(* Logix 5000 AddOnInstructionDefinition export SPEL_XYLimSet; software revision 30.01 *)

ADD_ON_INSTRUCTION SPEL_ExecCmd   (* revision 1.2 *)
// Executes a command in the robot controller.  Normally this is called by higher level AOIs.
VAR_INPUT
   Start : BOOL; {required}
   MaxTime : DINT := 3000; {required}
END_VAR
VAR_OUTPUT
   InCycle : BOOL; {access Read Only, visible}
   Done : BOOL; {access Read Only, visible}
   Error : BOOL; {access Read Only, visible}
END_VAR
VAR_IN_OUT
   ExtInputs : AB:ETHERNET_MODULE_INT_128Bytes:I:0; {required}
        .DATA[0].0   // ExtCmdGet
        .DATA[0].1   // ExtRespSet
        .DATA[0].2   // ExtCmdResult
        .DATA[0].3   // ExtError
   ExtOutputs : AB:ETHERNET_MODULE_INT_128Bytes:O:0; {required}
        .DATA[0].0   // ExtCmdSet
        .DATA[0].1   // ExtRespGet
        .DATA[0].2   // ExtCmdReset
END_VAR
VAR_INPUT
   Cmd : INT; {required}
   CmdParam1 : INT; {required}
   CmdParam2 : INT; {required}
   CmdParam3 : INT; {required}
   CmdParam4 : INT; {required}
   CmdParam5 : INT; {required}
   CmdParam6 : INT; {required}
   CmdParam7 : INT; {required}
END_VAR
VAR_OUTPUT
   CmdEcho : INT; {access Read Only, visible}
   Resp1 : INT; {access Read Only, visible}
   Resp2 : INT; {access Read Only, visible}
   Resp3 : INT; {access Read Only, visible}
   Resp4 : INT; {access Read Only, visible}
   Resp5 : INT; {access Read Only, visible}
   Resp6 : INT; {access Read Only, visible}
   Resp7 : INT; {access Read Only, visible}
   ErrCode1 : INT; {access Read Only, visible}
   ErrCode2 : INT; {access Read Only, visible}
END_VAR
VAR
   ExtReset : BOOL; {access None}
   ExtError : BOOL; {access None}
   ExtCmdSet : BOOL; {access None}   // Cmd Ready
   ExtCmdGet : BOOL; {access None}   // Cmd Received
   CmdXferDone : BOOL; {access None}
   ExtRespSet : BOOL; {access None}   // Resp Ready
   RespXferDone : BOOL; {access None}
   ExtCmdResult : BOOL; {access None}   // Normal or Error?
   TmrCmdDataRdy : TIMER := (PRE := 5); {access None}
   OneShotDoneOff : BOOL; {access None}
   OneShotStart : BOOL; {access None}
   StartInit : BOOL; {access None}
   OneShotStartError : BOOL; {access None}
   TmrCycle : TIMER := (PRE := 5000); {access None}
   OneshotTmrPreset : BOOL; {access None}
   TmrCmdSet : TIMER := (PRE := 20); {access None}
   OnShotCmdDataXfer : BOOL; {access None}
   OneShotRespDataXfer : BOOL; {access None}
   OneShotDataRdy : BOOL; {access None}
   OtherCmdInCycle : BOOL; {access None}
   s : BOOL; {access None}
   OneShotUnsetCmdIncycle : BOOL; {access None}
   OneShotSetCmdIncycle : BOOL; {access None}
   OneShotSetOtherCmdInCycleError : BOOL; {access None}
   OneShotSetBit : BOOL; {access None}
   MaxTimeError : BOOL; {access None}
END_VAR

ROUTINE Logic   (* ladder *)
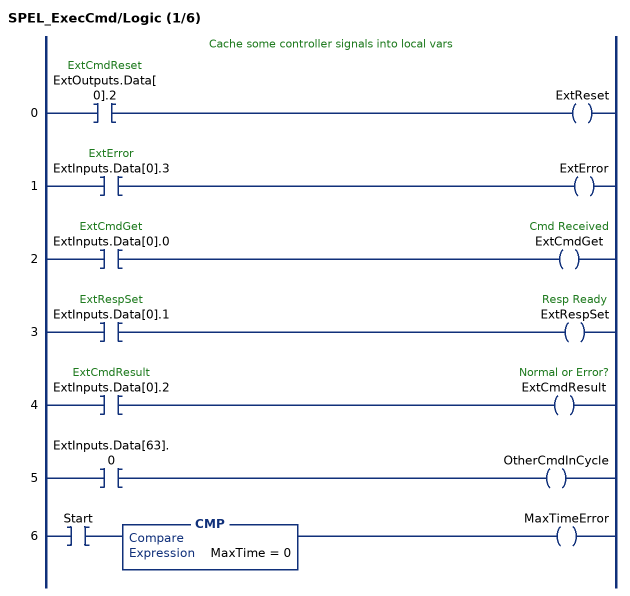
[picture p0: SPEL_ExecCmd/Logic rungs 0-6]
   // Cache some controller signals into local vars
   0: XIC(ExtOutputs.Data[0].2)OTE(ExtReset);
   1: XIC(ExtInputs.Data[0].3)OTE(ExtError);
   2: XIC(ExtInputs.Data[0].0)OTE(ExtCmdGet);
   3: XIC(ExtInputs.Data[0].1)OTE(ExtRespSet);
   4: XIC(ExtInputs.Data[0].2)OTE(ExtCmdResult);
   5: XIC(ExtInputs.Data[63].0)OTE(OtherCmdInCycle);
   6: XIC(Start)CMP(MaxTime = 0)OTE(MaxTimeError);
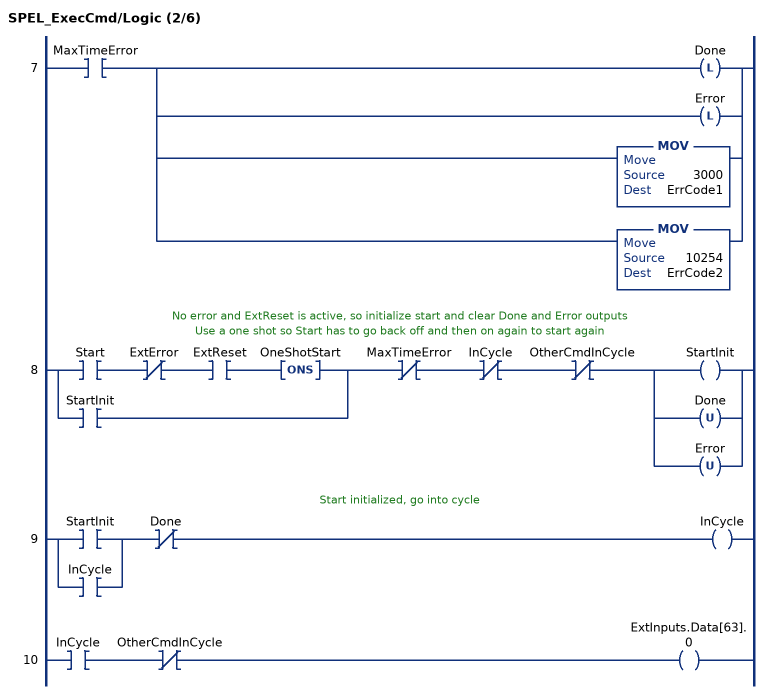
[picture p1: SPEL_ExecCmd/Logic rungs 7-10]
   7: XIC(MaxTimeError)[OTL(Done) ,OTL(Error) ,MOV(3000,ErrCode1) ,MOV(10254,ErrCode2) ];
   // No error and ExtReset is active, so initialize start and clear Done and Error outputs
   // Use a one shot so Start has to go back off and then on again to start again
   8: [XIC(Start) XIO(ExtError) XIC(ExtReset) ONS(OneShotStart) ,XIC(StartInit) ]XIO(MaxTimeError)XIO(InCycle)XIO(OtherCmdInCycle)[OTE(StartInit) ,OTU(Done) ,OTU(Error) ];
   // Start initialized, go into cycle
   9: [XIC(StartInit) ,XIC(InCycle) ]XIO(Done)OTE(InCycle);
   10: XIC(InCycle)XIO(OtherCmdInCycle)OTE(ExtInputs.Data[63].0);
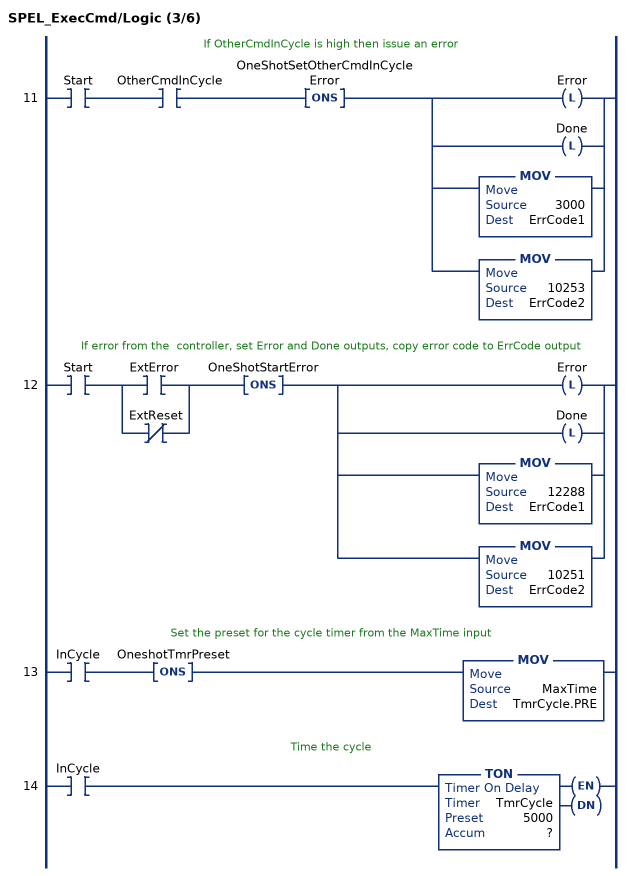
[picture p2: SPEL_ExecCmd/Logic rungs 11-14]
   // If OtherCmdInCycle is high then issue an error
   11: XIC(Start)XIC(OtherCmdInCycle)ONS(OneShotSetOtherCmdInCycleError)[OTL(Error) ,OTL(Done) ,MOV(3000,ErrCode1) ,MOV(10253,ErrCode2) ];
   // If error from the  controller, set Error and Done outputs, copy error code to ErrCode output
   12: XIC(Start)[XIC(ExtError) ,XIO(ExtReset) ]ONS(OneShotStartError)[OTL(Error) ,OTL(Done) ,MOV(12288,ErrCode1) ,MOV(10251,ErrCode2) ];
   // Set the preset for the cycle timer from the MaxTime input
   13: XIC(InCycle)ONS(OneshotTmrPreset)MOV(MaxTime,TmrCycle.PRE);
   // Time the cycle
   14: XIC(InCycle)TON(TmrCycle,?,?);
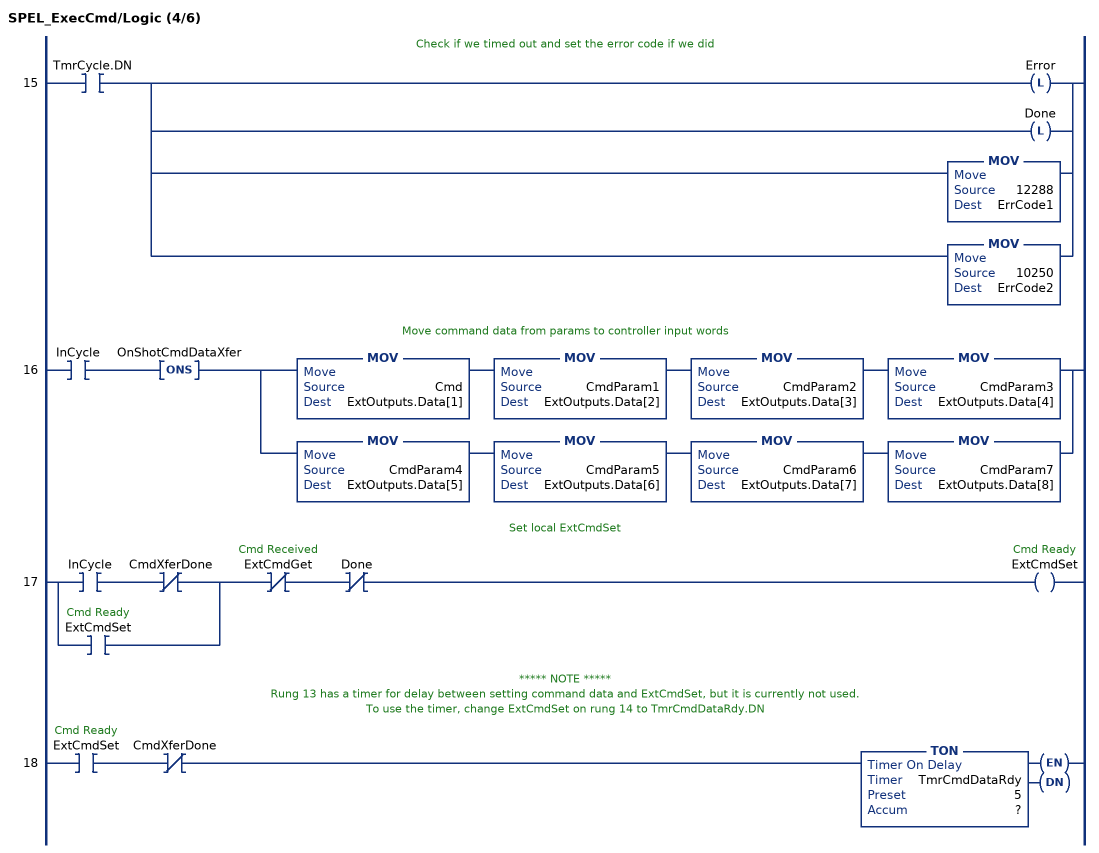
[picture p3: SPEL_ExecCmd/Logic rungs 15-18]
   // Check if we timed out and set the error code if we did
   15: XIC(TmrCycle.DN)[OTL(Error) ,OTL(Done) ,MOV(12288,ErrCode1) ,MOV(10250,ErrCode2) ];
   // Move command data from params to controller input words
   16: XIC(InCycle)ONS(OnShotCmdDataXfer)[MOV(Cmd,ExtOutputs.Data[1]) MOV(CmdParam1,ExtOutputs.Data[2]) MOV(CmdParam2,ExtOutputs.Data[3]) MOV(CmdParam3,ExtOutputs.Data[4]) ,MOV(CmdParam4,ExtOutputs.Data[5]) MOV(CmdParam5,ExtOutputs.Data[6]) MOV(CmdParam6,ExtOutputs.Data[7]) MOV(CmdParam7,ExtOutputs.Data[8]) ];
   // Set local ExtCmdSet
   17: [XIC(InCycle) XIO(CmdXferDone) ,XIC(ExtCmdSet) ]XIO(ExtCmdGet)XIO(Done)OTE(ExtCmdSet);
   // ***** NOTE *****
   // Rung 13 has a timer for delay between setting command data and ExtCmdSet, but it is currently not used.
   // To use the timer, change ExtCmdSet on rung 14 to TmrCmdDataRdy.DN
   18: XIC(ExtCmdSet)XIO(CmdXferDone)TON(TmrCmdDataRdy,?,?);
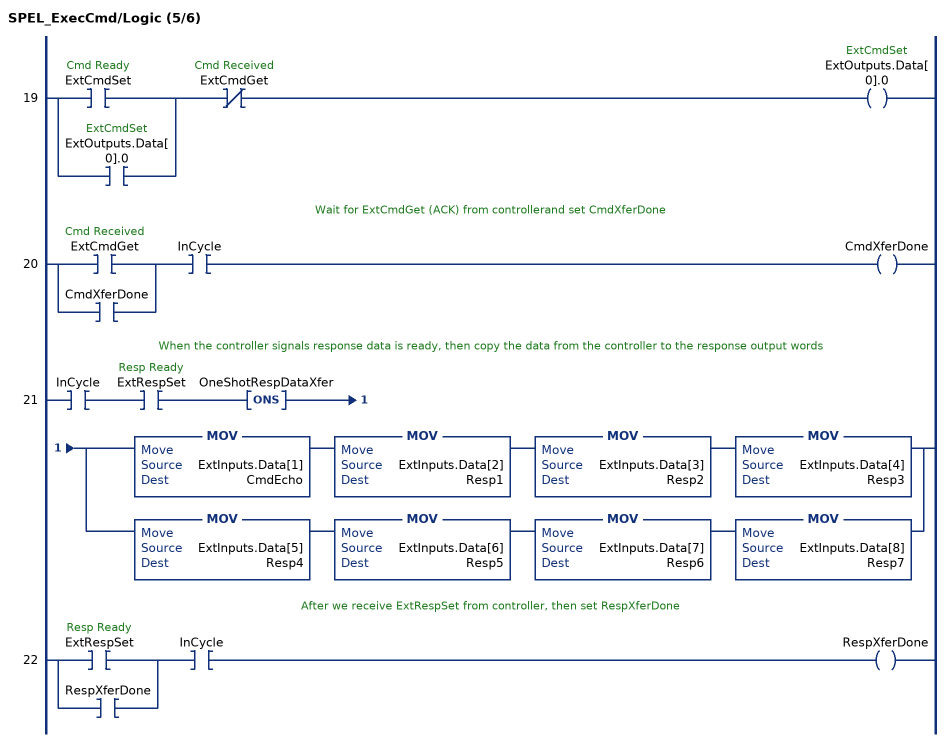
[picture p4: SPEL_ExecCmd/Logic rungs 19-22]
   19: [XIC(ExtCmdSet) ,XIC(ExtOutputs.Data[0].0) ]XIO(ExtCmdGet)OTE(ExtOutputs.Data[0].0);
   // Wait for ExtCmdGet (ACK) from controllerand set CmdXferDone
   20: [XIC(ExtCmdGet) ,XIC(CmdXferDone) ]XIC(InCycle)OTE(CmdXferDone);
   // When the controller signals response data is ready, then copy the data from the controller to the response output words
   21: XIC(InCycle)XIC(ExtRespSet)ONS(OneShotRespDataXfer)[MOV(ExtInputs.Data[1],CmdEcho) MOV(ExtInputs.Data[2],Resp1) MOV(ExtInputs.Data[3],Resp2) MOV(ExtInputs.Data[4],Resp3) ,MOV(ExtInputs.Data[5],Resp4) MOV(ExtInputs.Data[6],Resp5) MOV(ExtInputs.Data[7],Resp6) MOV(ExtInputs.Data[8],Resp7) ];
   // After we receive ExtRespSet from controller, then set RespXferDone
   22: [XIC(ExtRespSet) ,XIC(RespXferDone) ]XIC(InCycle)OTE(RespXferDone);
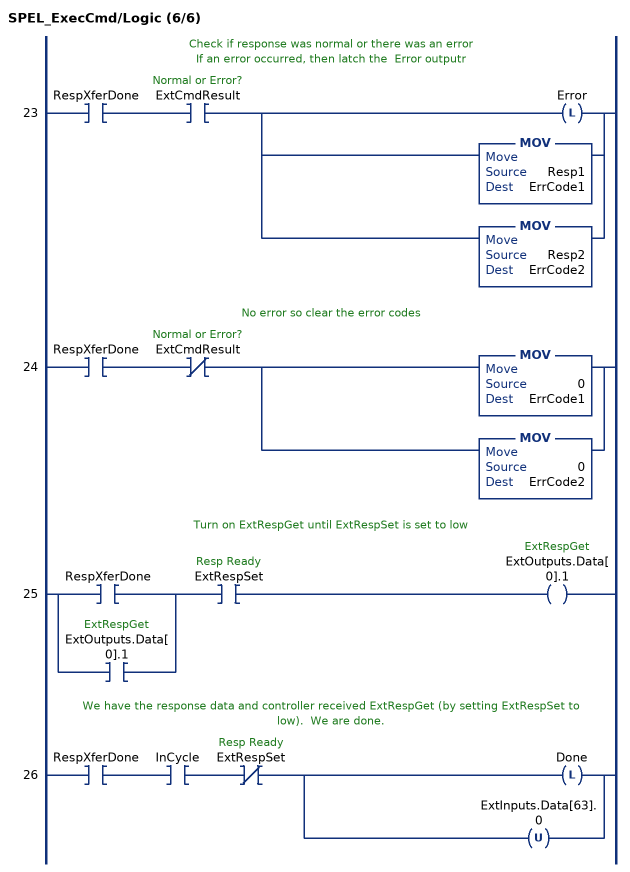
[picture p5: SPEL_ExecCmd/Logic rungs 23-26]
   // Check if response was normal or there was an error
   // If an error occurred, then latch the  Error outputr
   23: XIC(RespXferDone)XIC(ExtCmdResult)[OTL(Error) ,MOV(Resp1,ErrCode1) ,MOV(Resp2,ErrCode2) ];
   // No error so clear the error codes
   24: XIC(RespXferDone)XIO(ExtCmdResult)[MOV(0,ErrCode1) ,MOV(0,ErrCode2) ];
   // Turn on ExtRespGet until ExtRespSet is set to low
   25: [XIC(RespXferDone) ,XIC(ExtOutputs.Data[0].1) ]XIC(ExtRespSet)OTE(ExtOutputs.Data[0].1);
   // We have the response data and controller received ExtRespGet (by setting ExtRespSet to low).  We are done.
   26: XIC(RespXferDone)XIC(InCycle)XIO(ExtRespSet)[OTL(Done) ,OTU(ExtInputs.Data[63].0) ];
END_ROUTINE
END_ADD_ON_INSTRUCTION

ADD_ON_INSTRUCTION SPEL_XYLimSet   (* revision 1.2, vendor SEIKO EPSON CORP. *)
// Sets the allowable motion area by specifying the
// lower and upper limit positions.
VAR_OUTPUT
   InCycle : BOOL; {access Read Only, visible}
   Done : BOOL; {access Read Only, visible}
   Error : BOOL; {access Read Only, visible}
END_VAR
VAR_INPUT
   Start : BOOL; {required}
   XLower : REAL; {access Read Only, required}
   XUpper : REAL; {access Read Only, required}
   YLower : REAL; {access Read Only, required}
   YUpper : REAL; {access Read Only, required}
   ZLower : REAL; {access Read Only, required}
   ZUpper : REAL; {access Read Only, required}
END_VAR
VAR_IN_OUT
   ExtInputs : AB:ETHERNET_MODULE_INT_128Bytes:I:0; {required}
   ExtOutputs : AB:ETHERNET_MODULE_INT_128Bytes:O:0; {required}
END_VAR
VAR_OUTPUT
   ErrCode1 : INT; {access Read Only, visible}
   ErrCode2 : INT; {access Read Only, visible}
END_VAR
VAR
   ExecXYLimSetZ : SPEL_ExecCmd := (MaxTime := 3000); {access None}
   ExecXYLimSetY : SPEL_ExecCmd := (MaxTime := 3000); {access None}
   ExecXYLimSetX : SPEL_ExecCmd := (MaxTime := 3000); {access None}
   upperLimit_INTS : INT[2]; {access None}
   StartInit : BOOL[32]; {access None}
   OneShotStart : BOOL[32]; {access None}
   lowerLimit_INTS : INT[2]; {access None}
   Lowerx1000 : DINT; {access None}
   Upperx1000 : DINT; {access None}
   ExecTimeout : DINT; {access None}
END_VAR

ROUTINE Logic   (* ladder *)
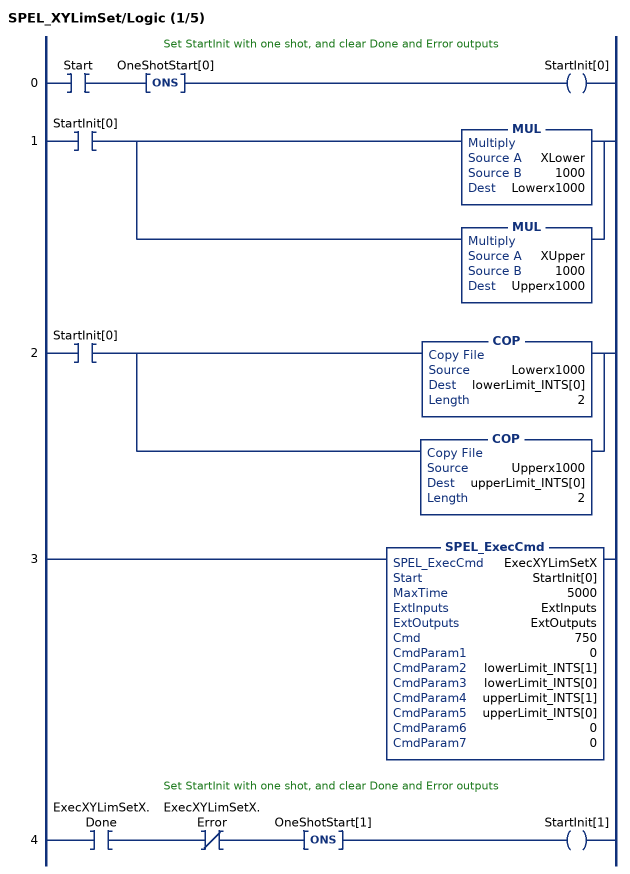
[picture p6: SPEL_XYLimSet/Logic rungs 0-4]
   // Set StartInit with one shot, and clear Done and Error outputs
   0: XIC(Start)ONS(OneShotStart[0])OTE(StartInit[0]);
   1: XIC(StartInit[0])[MUL(XLower,1000,Lowerx1000) ,MUL(XUpper,1000,Upperx1000) ];
   2: XIC(StartInit[0])[COP(Lowerx1000,lowerLimit_INTS[0],2) ,COP(Upperx1000,upperLimit_INTS[0],2) ];
   3: SPEL_ExecCmd(ExecXYLimSetX,StartInit[0],5000,ExtInputs,ExtOutputs,750,0,lowerLimit_INTS[1],lowerLimit_INTS[0],upperLimit_INTS[1],upperLimit_INTS[0],0,0);
   // Set StartInit with one shot, and clear Done and Error outputs
   4: XIC(ExecXYLimSetX.Done)XIO(ExecXYLimSetX.Error)ONS(OneShotStart[1])OTE(StartInit[1]);
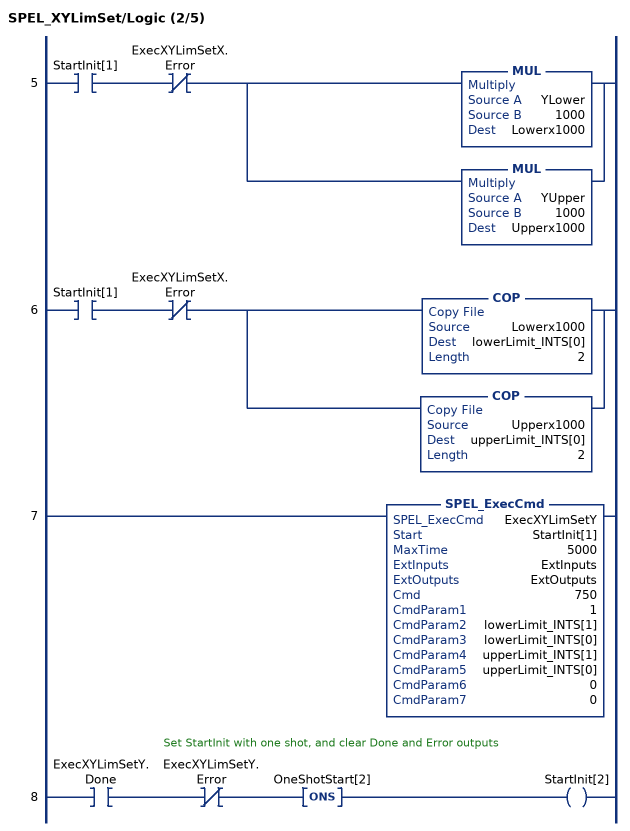
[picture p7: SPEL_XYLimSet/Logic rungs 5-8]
   5: XIC(StartInit[1])XIO(ExecXYLimSetX.Error)[MUL(YLower,1000,Lowerx1000) ,MUL(YUpper,1000,Upperx1000) ];
   6: XIC(StartInit[1])XIO(ExecXYLimSetX.Error)[COP(Lowerx1000,lowerLimit_INTS[0],2) ,COP(Upperx1000,upperLimit_INTS[0],2) ];
   7: SPEL_ExecCmd(ExecXYLimSetY,StartInit[1],5000,ExtInputs,ExtOutputs,750,1,lowerLimit_INTS[1],lowerLimit_INTS[0],upperLimit_INTS[1],upperLimit_INTS[0],0,0);
   // Set StartInit with one shot, and clear Done and Error outputs
   8: XIC(ExecXYLimSetY.Done)XIO(ExecXYLimSetY.Error)ONS(OneShotStart[2])OTE(StartInit[2]);
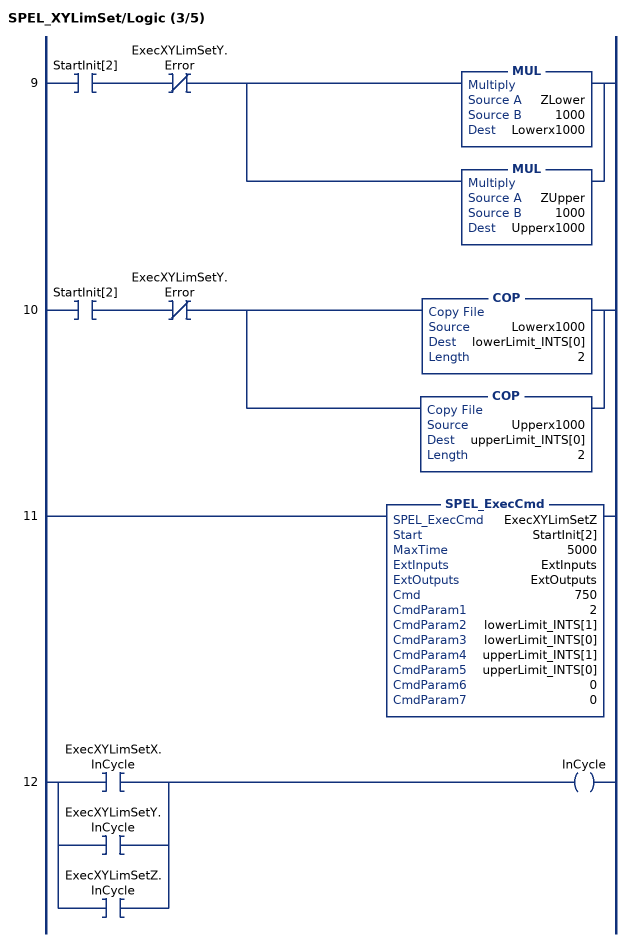
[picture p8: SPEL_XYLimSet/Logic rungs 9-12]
   9: XIC(StartInit[2])XIO(ExecXYLimSetY.Error)[MUL(ZLower,1000,Lowerx1000) ,MUL(ZUpper,1000,Upperx1000) ];
   10: XIC(StartInit[2])XIO(ExecXYLimSetY.Error)[COP(Lowerx1000,lowerLimit_INTS[0],2) ,COP(Upperx1000,upperLimit_INTS[0],2) ];
   11: SPEL_ExecCmd(ExecXYLimSetZ,StartInit[2],5000,ExtInputs,ExtOutputs,750,2,lowerLimit_INTS[1],lowerLimit_INTS[0],upperLimit_INTS[1],upperLimit_INTS[0],0,0);
   12: [XIC(ExecXYLimSetX.InCycle) ,XIC(ExecXYLimSetY.InCycle) ,XIC(ExecXYLimSetZ.InCycle) ]OTE(InCycle);
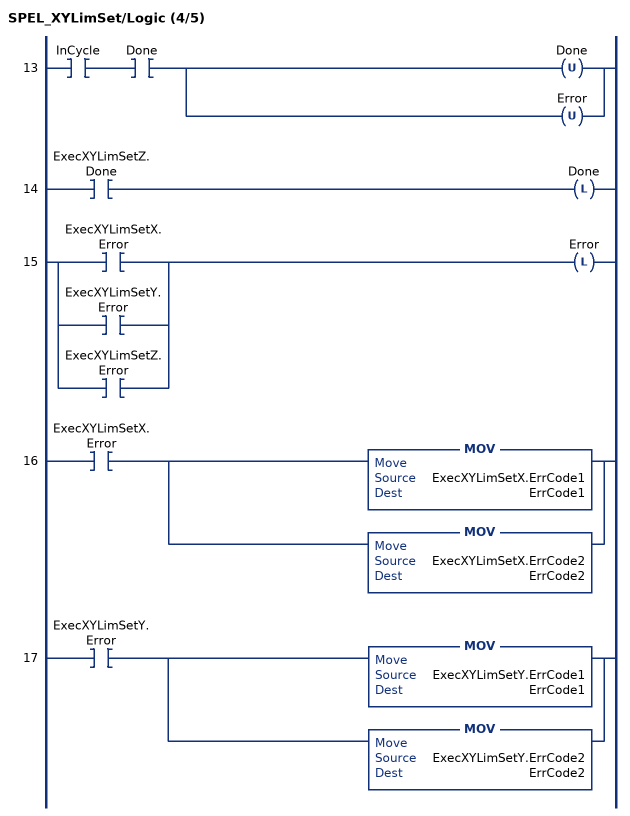
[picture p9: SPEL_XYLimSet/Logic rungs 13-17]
   13: XIC(InCycle)XIC(Done)[OTU(Done) ,OTU(Error) ];
   14: XIC(ExecXYLimSetZ.Done)OTL(Done);
   15: [XIC(ExecXYLimSetX.Error) ,XIC(ExecXYLimSetY.Error) ,XIC(ExecXYLimSetZ.Error) ]OTL(Error);
   16: XIC(ExecXYLimSetX.Error)[MOV(ExecXYLimSetX.ErrCode1,ErrCode1) ,MOV(ExecXYLimSetX.ErrCode2,ErrCode2) ];
   17: XIC(ExecXYLimSetY.Error)[MOV(ExecXYLimSetY.ErrCode1,ErrCode1) ,MOV(ExecXYLimSetY.ErrCode2,ErrCode2) ];
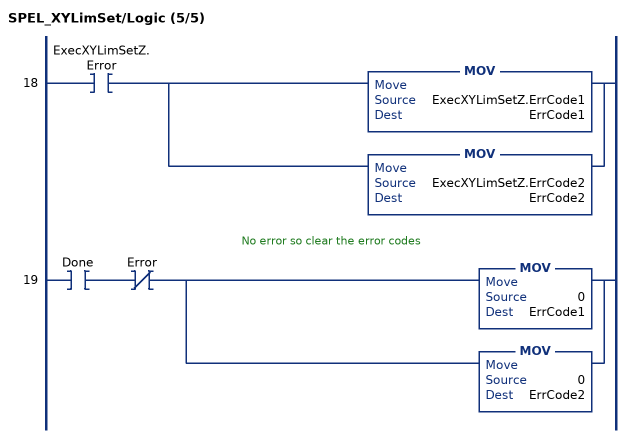
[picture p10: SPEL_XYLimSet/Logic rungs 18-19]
   18: XIC(ExecXYLimSetZ.Error)[MOV(ExecXYLimSetZ.ErrCode1,ErrCode1) ,MOV(ExecXYLimSetZ.ErrCode2,ErrCode2) ];
   // No error so clear the error codes
   19: XIC(Done)XIO(Error)[MOV(0,ErrCode1) ,MOV(0,ErrCode2) ];
END_ROUTINE
END_ADD_ON_INSTRUCTION
